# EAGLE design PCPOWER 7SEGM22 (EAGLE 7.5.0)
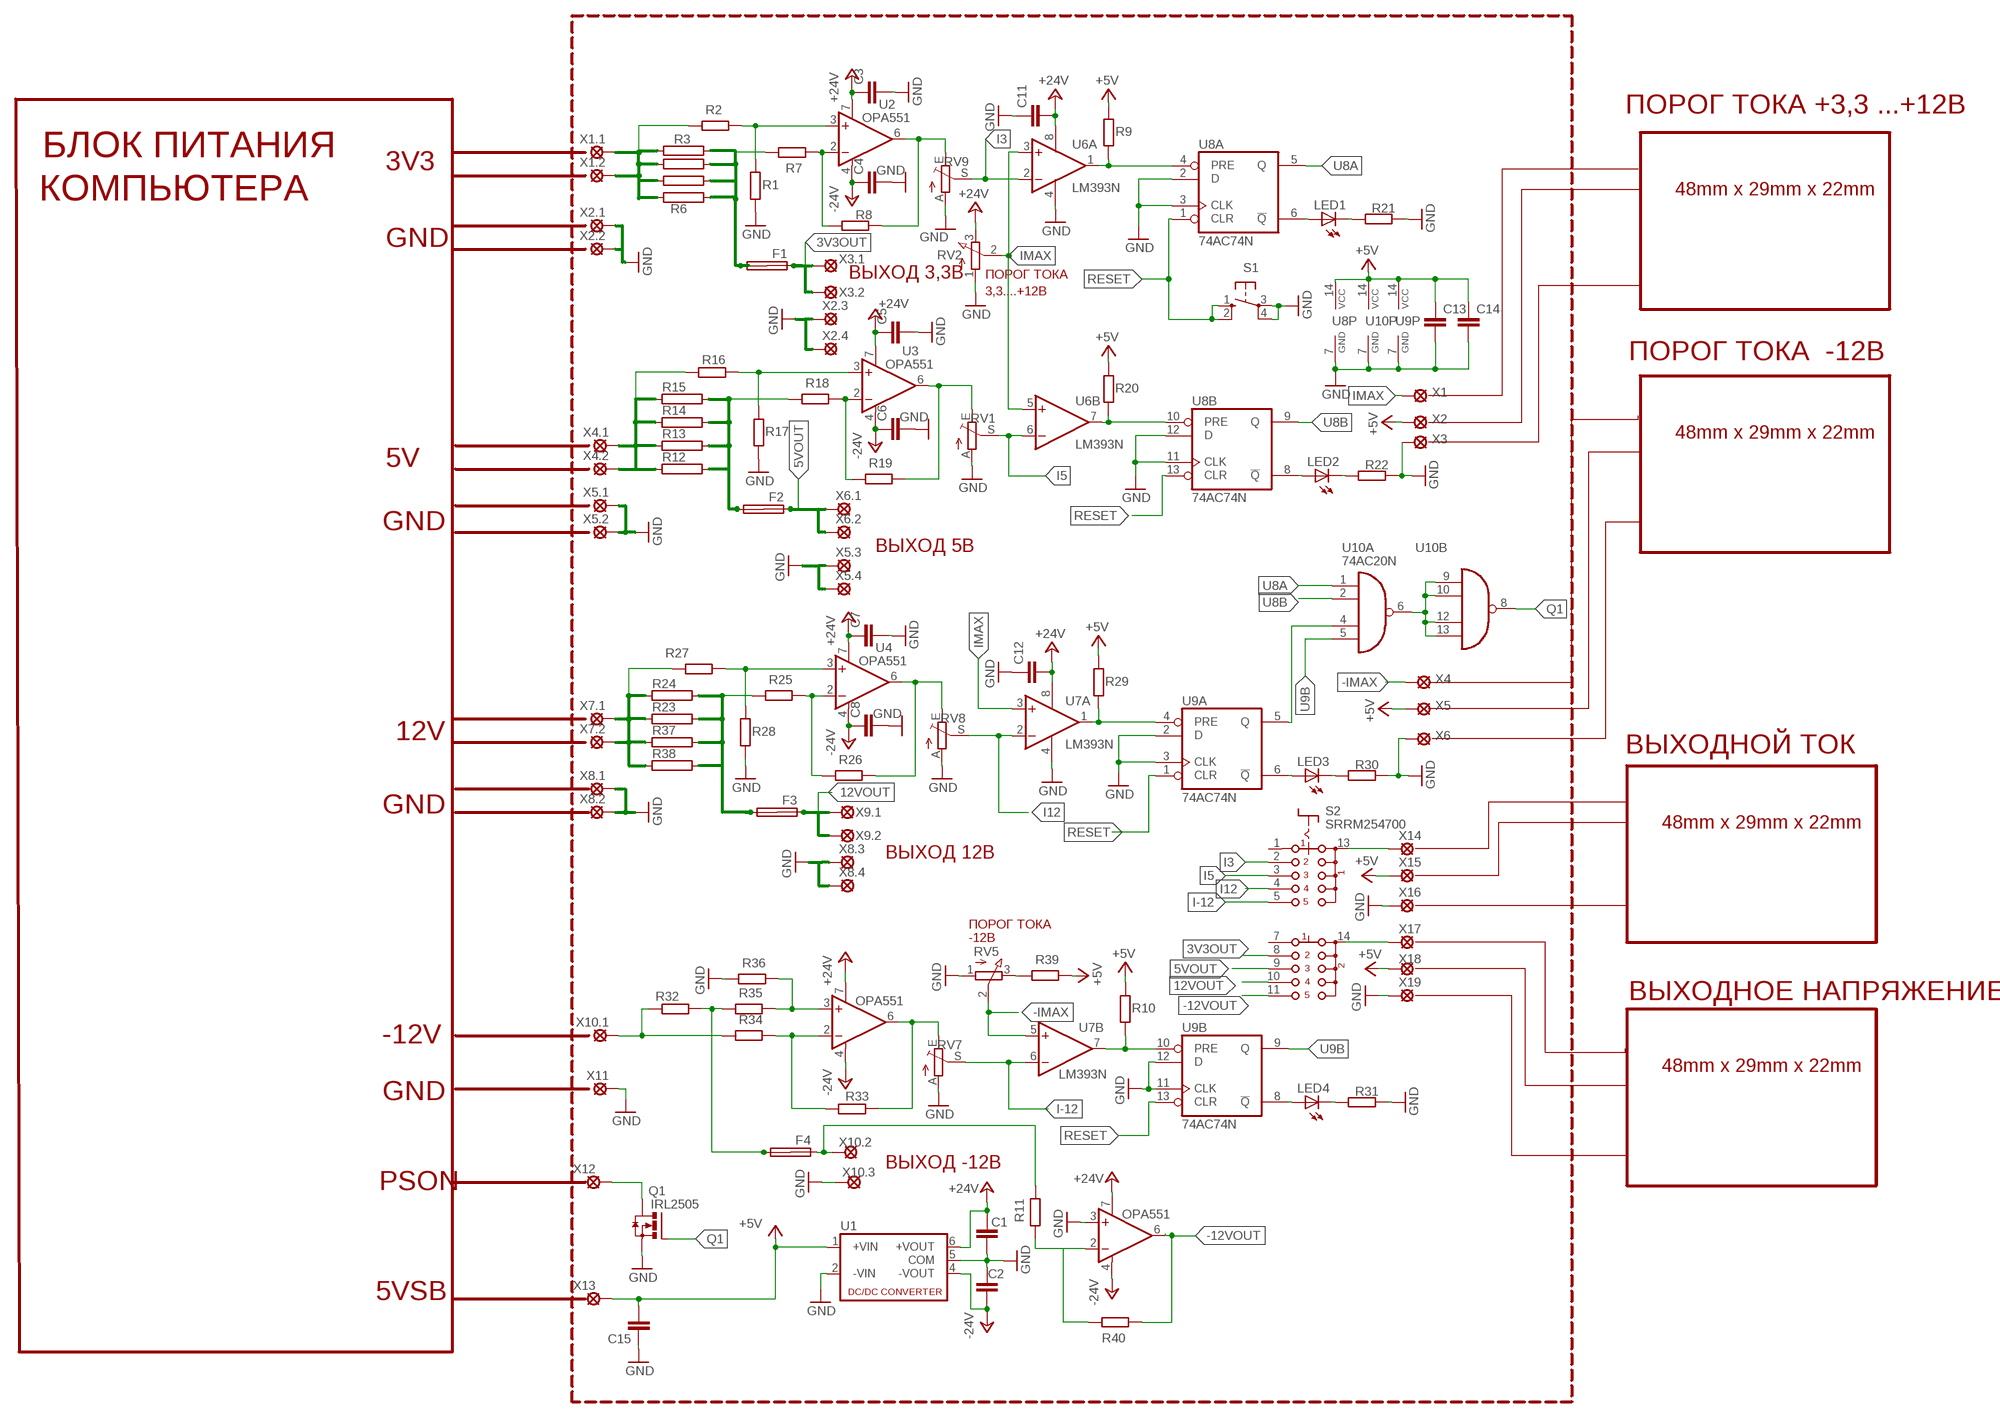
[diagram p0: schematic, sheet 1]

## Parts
C1  C-EUC1206  [C1206]
C2  C-EUC1206  [C1206]
C3  C-EUC1206  [C1206]
C4  C-EUC1206  [C1206]
C5  C-EUC1206  [C1206]
C6  C-EUC1206  [C1206]
C7  C-EUC1206  [C1206]
C8  C-EUC1206  [C1206]
C11  C-EUC1206  [C1206]
C12  C-EUC1206  [C1206]
C13  C-EUC1206  [C1206]
C14  C-EUC1206  [C1206]
C15  C-EUC1206  [C1206]
F1  SHK20L  [SHK20L]
F2  SHK20L  [SHK20L]
F3  SHK20L  [SHK20L]
F4  SHK20L  [SHK20L]
LED1  LED5MM  [LED5MM]
LED2  LED5MM  [LED5MM]
LED3  LED5MM  [LED5MM]
LED4  LED5MM  [LED5MM]
Q1  IRL2505  IRF3704L-V  [TO262-V]
R1  R-EU_0204/7  [0204/7]
R2  R-EU_0204/7  [0204/7]
R3  RKH208-8  [KH208-8]
R4  RKH208-8  [KH208-8]
R5  RKH208-8  [KH208-8]
R6  RKH208-8  [KH208-8]
R7  R-EU_0204/7  [0204/7]
R8  R-EU_0204/7  [0204/7]
R9  R-EU_0204/7  [0204/7]
R10  R-EU_0204/7  [0204/7]
R11  R-EU_0204/7  [0204/7]
R12  RKH208-8  [KH208-8]
R13  RKH208-8  [KH208-8]
R14  RKH208-8  [KH208-8]
R15  RKH208-8  [KH208-8]
R16  R-EU_0204/7  [0204/7]
R17  R-EU_0204/7  [0204/7]
R18  R-EU_0204/7  [0204/7]
R19  R-EU_0204/7  [0204/7]
R20  R-EU_0204/7  [0204/7]
R21  R-EU_0204/7  [0204/7]
R22  R-EU_0204/7  [0204/7]
R23  RKH208-8  [KH208-8]
R24  RKH208-8  [KH208-8]
R25  R-EU_0204/7  [0204/7]
R26  R-EU_0204/7  [0204/7]
R27  R-EU_0204/7  [0204/7]
R28  R-EU_0204/7  [0204/7]
R29  R-EU_0204/7  [0204/7]
R30  R-EU_0204/7  [0204/7]
R31  R-EU_0204/7  [0204/7]
R32  R-EU_0617/22  [0617/22]
R33  R-EU_0204/7  [0204/7]
R34  R-EU_0204/7  [0204/7]
R35  R-EU_0204/7  [0204/7]
R36  R-EU_0204/7  [0204/7]
R37  RKH208-8  [KH208-8]
R38  RKH208-8  [KH208-8]
R39  R-EU_0204/7  [0204/7]
R40  R-EU_0204/7  [0204/7]
RV1  TRIM_EU-CT6  [CT6]
RV2  PV09A  [PTV09]
RV5  PV09A  [PTV09]
RV7  TRIM_EU-CT6  [CT6]
RV8  TRIM_EU-CT6  [CT6]
RV9  TRIM_EU-CT6  [CT6]
S1  10-XX  [B3F-10XX]
S2  SRRM254700  [SRRM254700]
U1  NMA  [NMA]
U2  OPA551  OPA336P  [DIL08]
U3  OPA551  OPA336P  [DIL08]
U4  OPA551  OPA336P  [DIL08]
U5  OPA551  OPA336P  [DIL08]
U6  LM393N  [DIL08]
U7  LM393N  [DIL08]
U8  74AC74N  [DIL14]
U9  74AC74N  [DIL14]
U10  74AC20N  [DIL14]
U11  OPA551  OPA336P  [DIL08]
X1  LSP10  [LSP10]
X1.1  SE14  [SE14]
X1.2  SE14  [SE14]
X2  LSP10  [LSP10]
X2.1  SE14  [SE14]
X2.2  SE14  [SE14]
X2.3  SE14  [SE14]
X2.4  SE14  [SE14]
X3  LSP10  [LSP10]
X3.1  SE14  [SE14]
X3.2  SE14  [SE14]
X4  LSP10  [LSP10]
X4.1  SE14  [SE14]
X4.2  SE14  [SE14]
X5  LSP10  [LSP10]
X5.1  SE14  [SE14]
X5.2  SE14  [SE14]
X5.3  SE14  [SE14]
X5.4  SE14  [SE14]
X6  LSP10  [LSP10]
X6.1  SE14  [SE14]
X6.2  SE14  [SE14]
X7.1  SE14  [SE14]
X7.2  SE14  [SE14]
X8.1  SE14  [SE14]
X8.2  SE14  [SE14]
X8.3  SE14  [SE14]
X8.4  SE14  [SE14]
X9.1  SE14  [SE14]
X9.2  SE14  [SE14]
X10.1  SE14  [SE14]
X10.2  SE14  [SE14]
X10.3  SE14  [SE14]
X11  SE14  [SE14]
X12  SE14  [SE14]
X13  SE14  [SE14]
X14  LSP10  [LSP10]
X15  LSP10  [LSP10]
X16  LSP10  [LSP10]
X17  LSP10  [LSP10]
X18  LSP10  [LSP10]
X19  LSP10  [LSP10]

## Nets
3V3OUT: F1.1A S2.8 X3.1.MP X3.2.MP
5VOUT: F2.1A S2.9 X6.1.MP X6.2.MP
12VOUT: F3.1A S2.10 X9.1.MP X9.2.MP
+5V: C13.1 C14.1 C15.2 R9.2 R10.2 R20.2 R29.2 R39.1 U1.1(+VIN) U8.14(P:VCC) U9.14(P:VCC) U10.14(P:VCC) X2.MP X5.MP X13.MP X15.MP X18.MP
+24V: C1.1 C3.1 C5.1 C7.1 C11.2 C12.2 RV2.3(E) U1.6(+VOUT) U2.7(V+) U3.7(V+) U4.7(V+) U5.7(V+) U6.8(P:V+) U7.8(P:V+) U11.7(V+)
-12VOUT: R40.2 S2.11
-24V: C2.2 C4.1 C6.1 C8.1 U1.4(-VOUT) U2.4(V-) U3.4(V-) U4.4(V-) U5.4(V-) U11.4(V-)
-IMAX: RV5.2(S) U7.5(B:+IN) X4.MP
GND: C1.2 C2.1 C3.2 C4.2 C5.2 C6.2 C7.2 C8.2 C11.1 C12.1 C13.2 C14.2 C15.1 Q1.3(S) R1.1 R17.1 R21.2 R22.2 R28.1 R30.2 R31.2 R36.2 RV1.A RV2.1(A) RV5.1(A) RV7.A RV8.A RV9.A S1.3(P) S1.4(P1) U1.2(-VIN) U1.5(COM) U6.4(P:V-) U7.4(P:V-) U8.2(A:D) U8.3(A:CLK) U8.7(P:GND) U8.11(B:CLK) U8.12(B:D) U9.2(A:D) U9.3(A:CLK) U9.7(P:GND) U9.11(B:CLK) U9.12(B:D) U10.7(P:GND) U11.3(+IN) X2.1.MP X2.2.MP X2.3.MP X2.4.MP X3.MP X5.1.MP X5.2.MP X5.3.MP X5.4.MP X6.MP X8.1.MP X8.2.MP X8.3.MP X8.4.MP X10.3.MP X11.MP X16.MP X19.MP
I3: RV9.S S2.2 U6.2(A:-IN)
I5: RV1.S S2.3 U6.6(B:-IN)
I12: RV8.S S2.4 U7.2(A:-IN)
I-12: RV7.S S2.5 U7.6(B:-IN)
IMAX: RV2.2(S) U6.3(A:+IN) U6.5(B:+IN) U7.3(A:+IN) X1.MP
N$1: R1.2 R2.1 U2.3(+IN)
N$2: R7.2 R8.1 U2.2(-IN)
N$3: R8.2 RV9.E U2.6(OUT)
N$4: R23.1 R24.1 R27.2 R37.1 R38.1 X7.1.MP X7.2.MP
N$5: R9.1 U6.1(A:OUT) U8.4(A:PRE)
N$6: R12.1 R13.1 R14.1 R15.1 R16.2 X4.1.MP X4.2.MP
N$7: F2.2A R12.2 R13.2 R14.2 R15.2 R18.2
N$8: R16.1 R17.2 U3.3(+IN)
N$9: R18.1 R19.2 U3.2(-IN)
N$10: R19.1 RV1.E U3.6(OUT)
N$11: F3.2A R23.2 R24.2 R25.2 R37.2 R38.2
N$12: R27.1 R28.2 U4.3(+IN)
N$13: R25.1 R26.2 U4.2(-IN)
N$14: R26.1 RV8.E U4.6(OUT)
N$15: R20.1 U6.7(B:OUT) U8.10(B:PRE)
N$16: R29.1 U7.1(A:OUT) U9.4(A:PRE)
N$17: R32.1 R34.2 X10.1.MP
N$18: R33.2 R34.1 U5.2(-IN)
N$19: R33.1 RV7.E U5.6(OUT)
N$20: F4.2A R32.2 R35.2
N$21: R35.1 R36.1 U5.3(+IN)
N$22: R39.2 RV5.3(E)
N$23: F4.1A R11.1 X10.2.MP
N$24: R10.1 U7.7(B:OUT) U9.10(B:PRE)
N$25: S2.13(C1) X14.MP
N$26: S2.14(C2) X17.MP
N$27: R11.2 R40.1 U11.2(-IN)
N$29: LED1.A U8.6(A:!Q)
N$30: LED1.K(C) R21.1
N$31: LED2.A U8.8(B:!Q)
N$32: LED2.K(C) R22.1
N$33: Q1.2(D) X12.MP
N$35: LED3.A U9.6(A:!Q)
N$37: LED3.K(C) R30.1
N$38: LED4.A U9.8(B:!Q)
N$39: LED4.K(C) R31.1
N$40: U9.5(A:Q) U10.4(A:I2)
N$42: U10.6(A:O) U10.9(B:I0) U10.10(B:I1) U10.12(B:I2) U10.13(B:I3)
N$44: F1.2A R3.2 R4.2 R5.2 R6.2 R7.1
N$45: R2.2 R3.1 R4.1 R5.1 R6.1 X1.1.MP X1.2.MP
Q1: Q1.1(G) U10.8(B:O)
RESET: S1.1(S) S1.2(S1) U8.1(A:CLR) U8.13(B:CLR) U9.1(A:CLR) U9.13(B:CLR)
U8A: U8.5(A:Q) U10.1(A:I0)
U8B: U8.9(B:Q) U10.2(A:I1)
U9B: U9.9(B:Q) U10.5(A:I3)
Unconnected: F1.1B F1.2B F2.1B F2.2B F3.1B F3.2B F4.1B F4.2B S2.1 S2.7 U11.6(OUT)

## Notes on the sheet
- ПОРОГ ТОКА +3,3 ...+12В
- БЛОК ПИТАНИЯ
- 3V3
- КОМПЬЮТЕРА | 48mm x 29mm x 22mm
- GND
- ВЫХОД 3,3В | ПОРОГ ТОКА
- 3,3....+12В
- ПОРОГ ТОКА  -12В
- 48mm x 29mm x 22mm
- 5V
- GND
- ВЫХОД 5В
- 12V
- ВЫХОДНОЙ ТОК
- GND
- 48mm x 29mm x 22mm
- ВЫХОД 12В
- ПОРОГ ТОКА
- -12В
- ВЫХОДНОЕ НАПРЯЖЕНИЕ
- -12V
- 48mm x 29mm x 22mm
- GND
- ВЫХОД -12В
- PSON
- 5VSB

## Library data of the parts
C1-C8 C11-C15 = rcl:C-EU: CAPACITOR, European symbol
F1-F4 = fuse:SHK20L: FUSE HOLDER 5 x 20 mm, SH contact, SHH1 Schukat, E1073 Buerklin; OC_FARNELL: unknown; OC_NEWARK: unknown
LED1-LED4 = led:LED: LED
Q1 = transistor-power:IRF3704: SMPS MOSFET HEXFET® Power MOSFET Source: http://www.irf.com/product-info/datasheets/data/irf3704.pdf
R1 R2 R7-R11 R16-R22 R25-R36 R39 R40 = rcl:R-EU_: RESISTOR, European symbol
R3-R6 R12-R15 R23 R24 R37 R38 = resistor-power:R: Power Resitor; OC_FARNELL: unknown; OC_NEWARK: unknown
RV1 RV7-RV9 = pot:TRIM_EU-: POTENTIOMETER
RV2 RV5 = pot:PV09A
S1 = switch-omron:10-XX: OMRON SWITCH; MPN: B3F-1000; OC_FARNELL: 176432; OC_NEWARK: 36M3542
S2 = switch:SRRM254700: 12-position General-purpose Vertical Type Rotary Switch 2 Pole 5 Positions Source: ALPS - SRRM.pdf
U1 = dc-dc-converter:NMA: DC-DC CONVERTER; MF: C & D TECHNOLOGIES, INC; MPN: NMA0515SC; OC_FARNELL: 1021434; OC_NEWARK: 61K3064
U2-U5 U11 = burr-brown:OPA336: CMOS Operational Amplifiers Single-Supply, MicroPower, MicroAmplifier(TM) Series; OC_FARNELL: unknown; OC_NEWARK: unknown
U6 U7 = linear:LM393: COMPARATOR
U8 U9 = 74xx-eu:74*74: Dual D type positive edge triggered FLIP FLOP, preset and clear
U10 = 74xx-eu:74*20: Dual 4-input NAND gate
X1-X6 X14-X19 = solpad:LSP10: SOLDER PAD
X1.1 X1.2 X2.1-X2.4 X3.1 X3.2 X4.1 X4.2 X5.1-X5.4 X6.1 X6.2 X7.1 X7.2 X8.1-X8.4 X9.1 X9.2 X10.1-X10.3 X11-X13 = solpad:SE14: SOLDER PAD

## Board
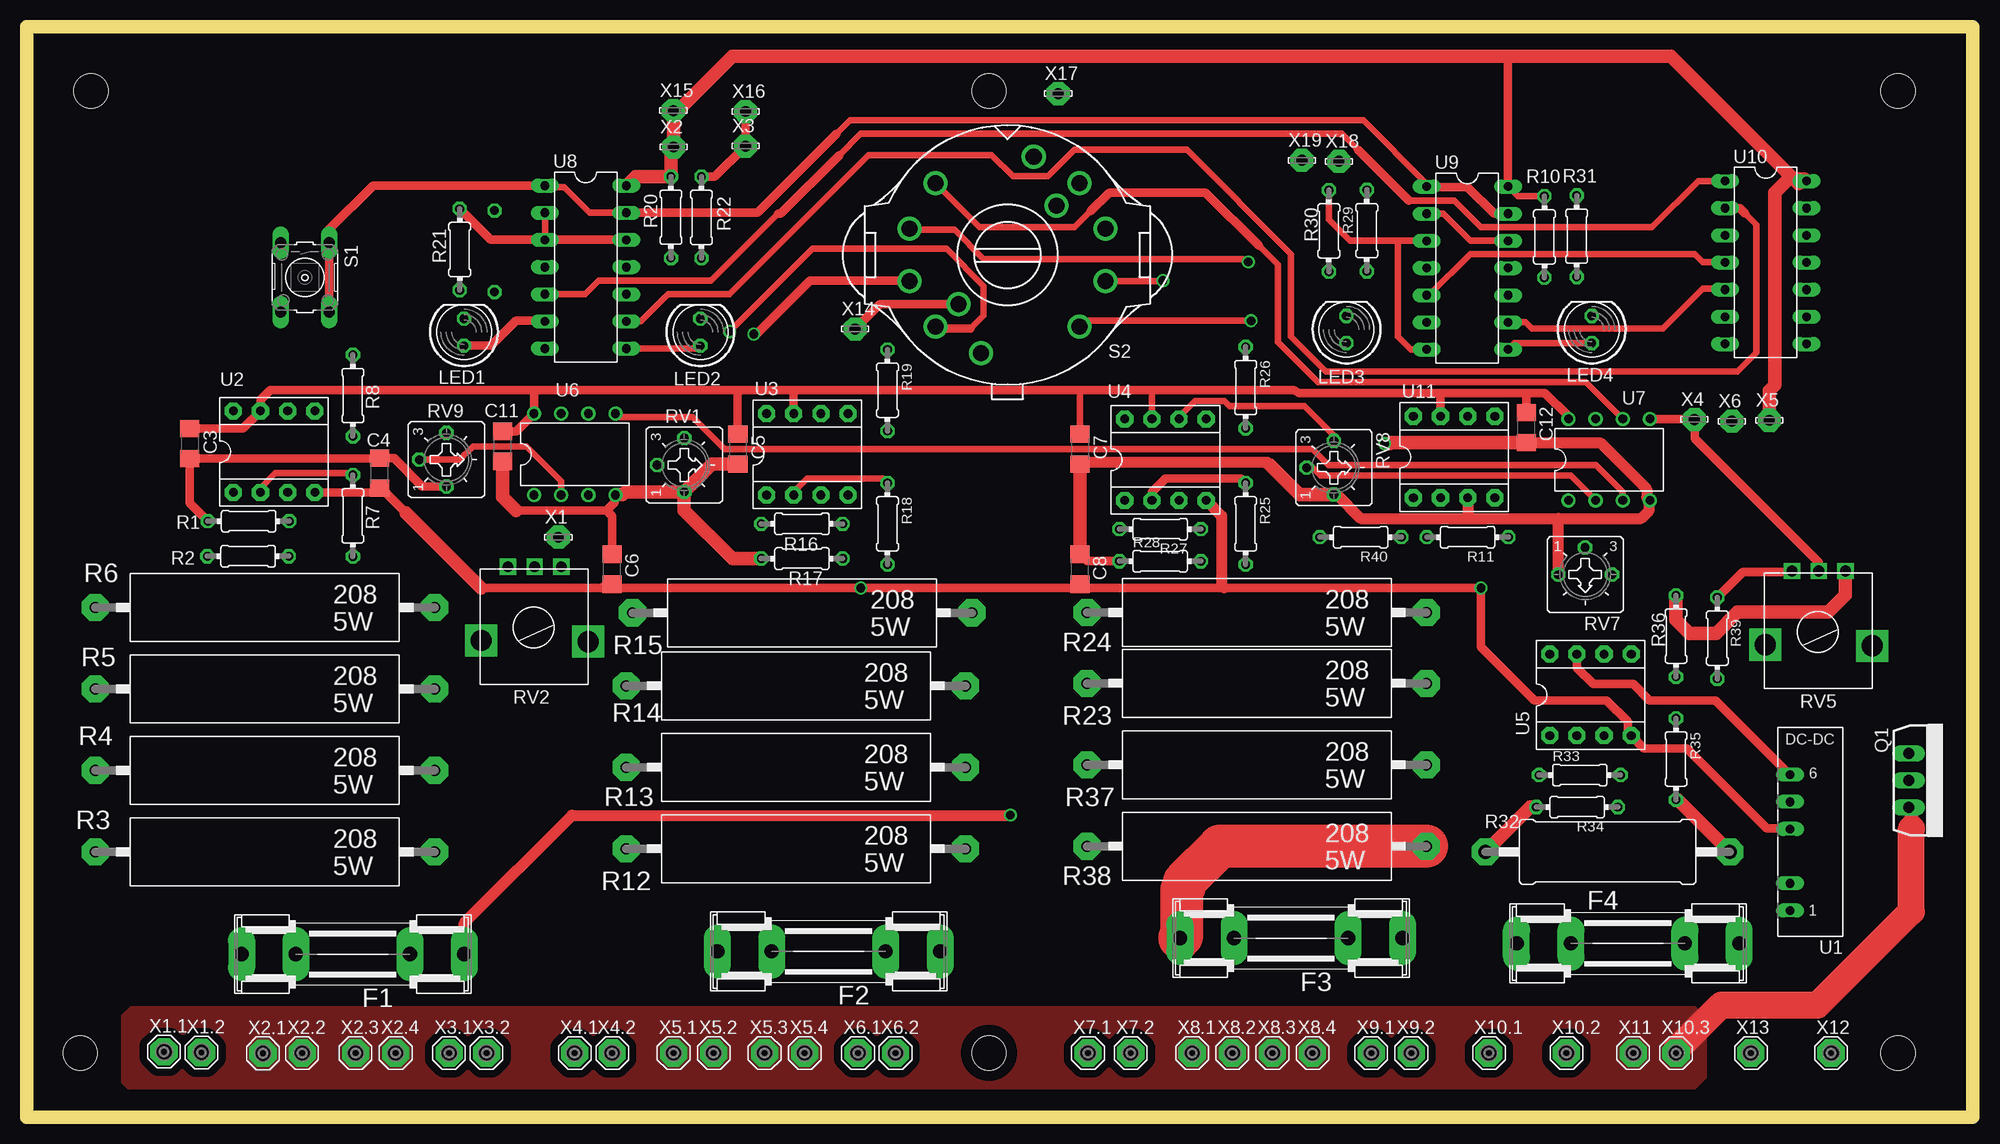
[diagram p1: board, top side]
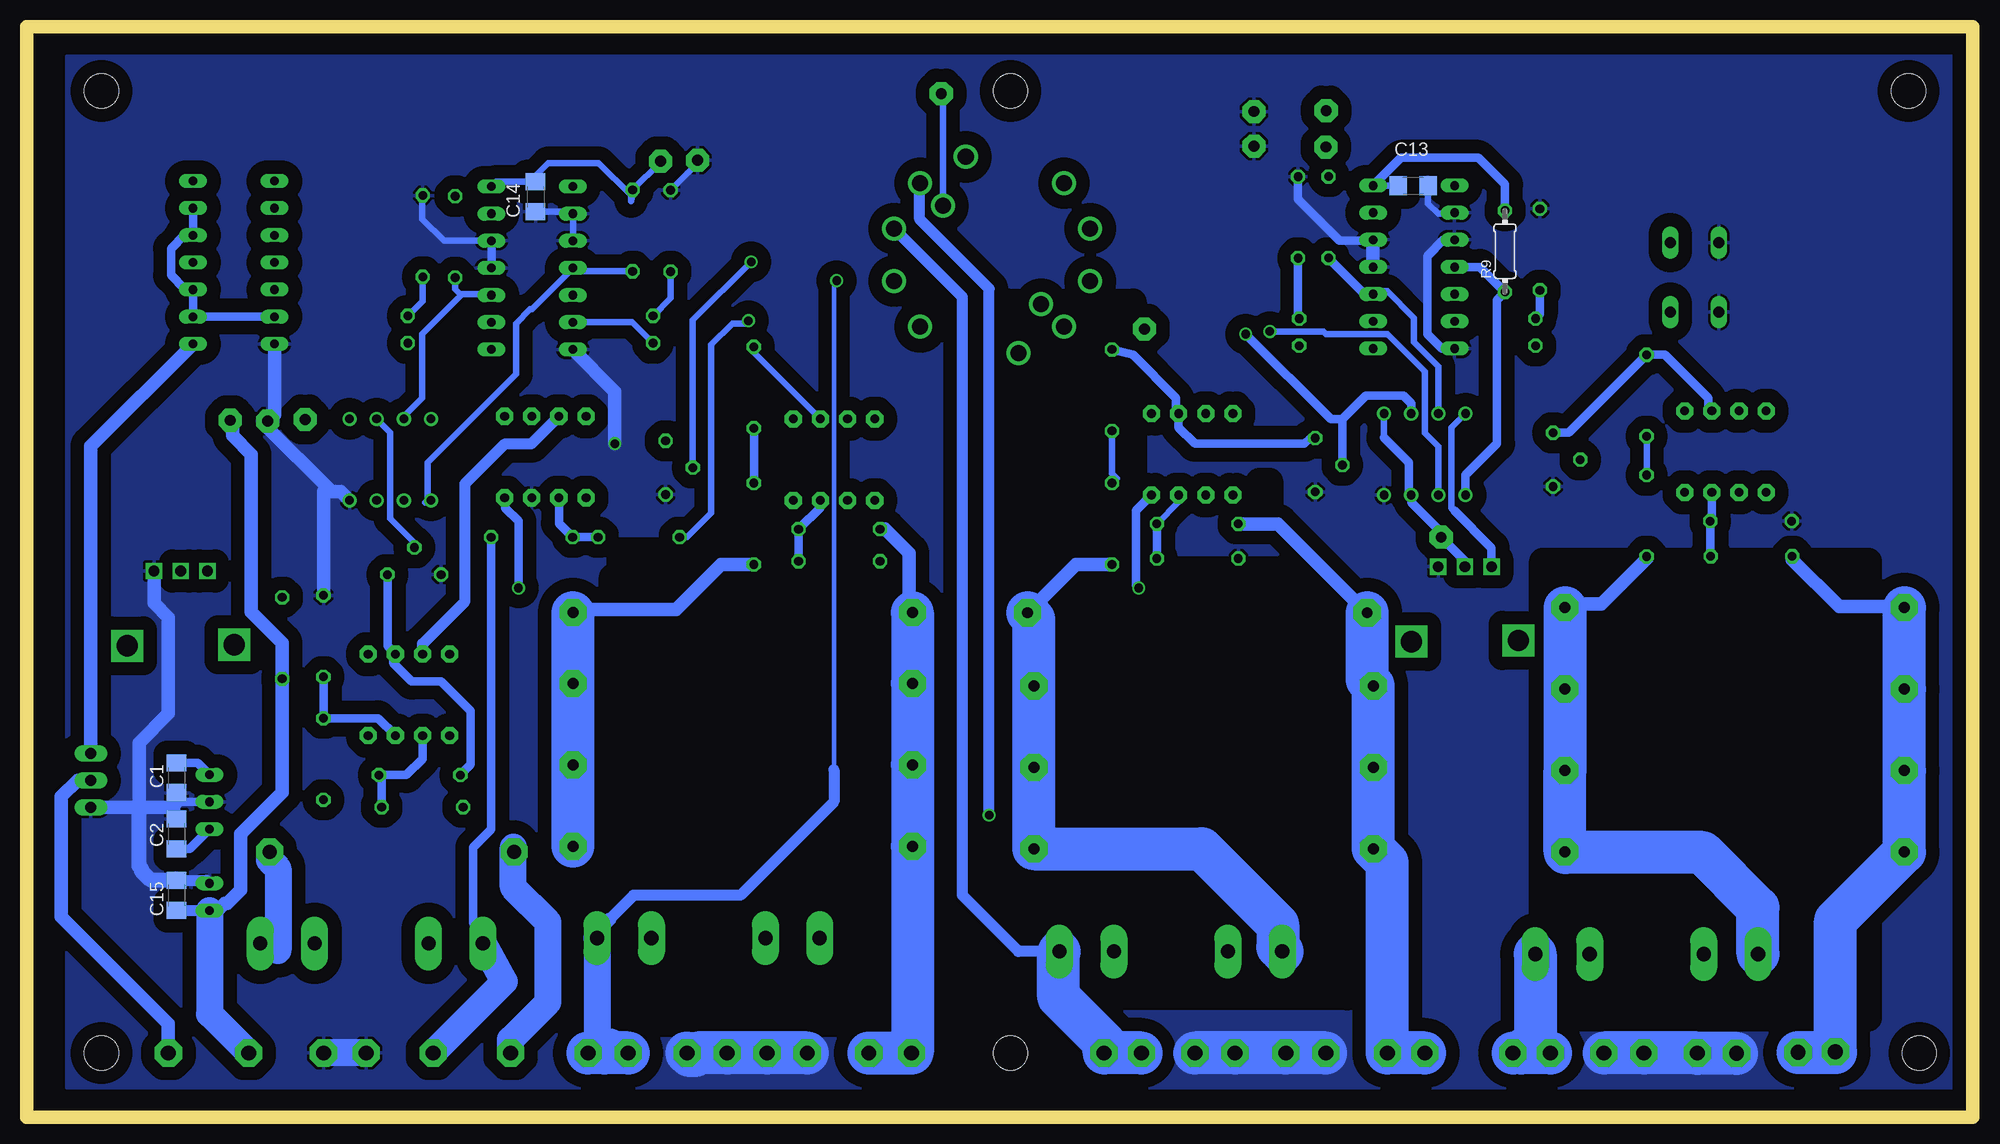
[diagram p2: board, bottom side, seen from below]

Size 182 x 102 mm. Coordinates in mm from the lower left corner, seen from the top.
Outline: 0,102 182,102 182,0 0,0 0,102
Copper layers (1*16): Top 0.035mm / dielectric 1.5mm / Bottom 0.035mm
Design rules "default": minimum track width 10mil, minimum drill 24mil, track to track 8mil, track to pad 8mil, pad to pad 8mil, via to via 8mil, smd to smd 8mil, copper to edge 40mil, drill to drill 8mil, minimum pad ring 10mil, minimum via ring 8mil, stop-mask expansion 4mil, vias tented up to drill 0mil, thermal gap 10mil
Holes 3.2 mm at 5,6 90,6 175,6 175,96 90,96 6,96
bRestrict: area 63.2,47 to 63.5,48.5; area 64.8,34 to 80.5,51.2; area 59.5,29 to 64.8,50.5; area 58.8,28.2 to 85.5,36; area 58.5,11.2 to 94,27.2; area 9.8,9.2 to 40.2,52; area 78.5,50.5 to 90.2,76.2; area 101.8,50.2 to 102,51.5; area 107.2,24 to 127.2,50.5; area 100,8.8 to 126.5,53; area 65.8,57.5 to 66.8,59.5

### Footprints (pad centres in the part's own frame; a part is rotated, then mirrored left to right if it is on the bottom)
C1206 = smd 1.6 x 1.8: 1 -1.4,0; 2 1.4,0
SHK20L = drill 1.321 pad 2.54 long: 1A -10.414,0; 1B -5.334,0; 2A 10.414,0; 2B 5.334,0
LED5MM = drill 0.813 octagon: A -1.27,0; K 1.27,0
TO262-V = drill 1.016 long: 1 -2.54,0; 2 0,0; 3 2.54,0
0204/7 = drill 0.813 octagon: 1 -3.81,0; 2 3.81,0
KH208-8 = drill 1.016 pad 2.54 octagon: 1 -15.875,0; 2 15.875,0
0617/22 = drill 1.3 pad 2.54 octagon: 1 -11.43,0; 2 11.43,0
CT6 = drill 0.813 octagon: A 2.515,0; E -2.515,0; S 0,-2.54
PTV09 = drill 1 square: 1 -2.5,0; 2 0,0; 3 2.5,0 | drill 2 square: P$4 -5,7; P$5 5,6.9
B3F-10XX = drill 1.016 long: 1 -3.251,2.261; 2 3.251,2.261; 3 -3.251,-2.261; 4 3.251,-2.261
SRRM254700 = drill 1.5 pad 2.184: 1 -9.176,2.459; 2 -6.718,6.718; 3 -2.459,9.176; 4 2.459,9.176; 5 6.718,6.718; 7 9.176,-2.459; 8 6.718,-6.718; 9 2.459,-9.176; 10 -2.459,-9.176; 11 -6.718,-6.718; 13 -4.596,4.596; 14 4.596,-4.596
NMA = drill 0.813 long: 1 0,6.35; 2 0,3.81; 4 0,-1.27; 5 0,-3.81; 6 0,-6.35
DIL08 = drill 0.813 pad 1.6 octagon: 1 -3.81,-3.81; 2 -1.27,-3.81; 3 1.27,-3.81; 4 3.81,-3.81; 5 3.81,3.81; 6 1.27,3.81; 7 -1.27,3.81; 8 -3.81,3.81
DIL08' = drill 0.813 pad 1.27: 1 -3.81,-3.81; 2 -1.27,-3.81; 3 1.27,-3.81; 4 3.81,-3.81; 5 3.81,3.81; 6 1.27,3.81; 7 -1.27,3.81; 8 -3.81,3.81
DIL14 = drill 0.813 long: 1 -7.62,-3.81; 2 -5.08,-3.81; 3 -2.54,-3.81; 4 0,-3.81; 5 2.54,-3.81; 6 5.08,-3.81; 7 7.62,-3.81; 8 7.62,3.81; 9 5.08,3.81; 10 2.54,3.81; 11 0,3.81; 12 -2.54,3.81; 13 -5.08,3.81; 14 -7.62,3.81
LSP10 = drill 1.016 pad 2.159 octagon: MP 0,0
SE14 = drill 1.397 pad 2.54 octagon: MP 0,0

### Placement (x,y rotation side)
C1  168,31.75 270 bottom
C2  168,26.5 270 bottom
C3  15.25,63 270 top
C4  33,60.25 90 top
C5  66.5,62.5 270 top
C6  54.75,51.25 90 top
C7  98.5,62.5 270 top
C8  98.5,51.25 90 top
C11  44.5,62.75 90 top
C12  140.25,64.5 90 top
C13  52.34,87.14 0 bottom
C14  134.42,86.09 270 bottom
C15  168,20.75 270 bottom
F1  30.5,15.25 180 top
F2  75,15.5 180 top
F3  118.25,16.75 180 top
F4  149.75,16.25 0 top
LED1  40.89,73.43 90 top
LED2  63,73.43 90 top
LED3  123.43,73.68 90 top
LED4  146.36,73.68 90 top
Q1  176,31.5 270 top
R1  20.75,55.75 0 top
R2  20.7,52.47 180 top
R3  22.27,24.81 0 top
R4  22.27,32.43 0 top
R5  22.27,40.05 0 top
R6  22.27,47.67 0 top
R7  30.5,56.25 90 top
R8  30.5,67.5 90 top
R9  43.75,81 90 bottom
R10  141.94,82.34 90 top
R11  134.75,54.25 180 top
R12  71.93,25.11 0 top
R13  71.93,32.73 0 top
R14  71.93,40.35 0 top
R15  72.52,47.18 0 top
R16  72.5,55.5 180 top
R17  72.5,52.25 0 top
R18  80.5,55.5 270 top
R19  80.5,68 270 top
R20  60.25,84.18 90 top
R21  40.49,81.16 90 top
R22  63.1,84.16 90 top
R23  115.04,40.58 0 top
R24  115.04,47.2 0 top
R25  114,55.5 270 top
R26  114,68.25 270 top
R27  106,55 180 top
R28  106,52 0 top
R29  125.33,82.93 90 top
R30  121.78,82.91 90 top
R31  144.96,82.41 90 top
R32  147.86,24.82 0 top
R33  145.25,32 0 top
R34  145,29 180 top
R35  154.25,33.5 270 top
R36  154.25,45 90 top
R37  115.04,32.96 0 top
R38  115.04,25.34 0 top
R39  158.11,44.81 90 top
R40  124.75,54.25 180 top
RV1  61.5,61 270 top
RV2  47.5,51.49 180 top
RV5  167.6,51.09 180 top
RV7  145.75,50.75 180 top
RV8  122.25,60.75 270 top
RV9  39.25,61.5 270 top
S1  26.02,78.55 270 top
S2  91.72,80.65 90 top
U1  164.91,25.68 180 top
U2  23.13,62.25 0 top
U3  73,62 0 top
U4  106.5,61.5 0 top
U5  146.25,39.5 0 top
U6  LM393N  [DIL08']  51.25,62 0 top
U7  LM393N  [DIL08']  148,61.5 0 top
U8  52.27,79.52 270 top
U9  134.73,79.43 270 top
U10  162.64,79.95 270 top
U11  133.5,61.75 0 top
X1  49.72,54.25 0 top
X1.1  12.84,6.13 0 top
X1.2  16.34,6.05 0 top
X2  60.5,90.75 0 top
X2.1  22.09,5.97 0 top
X2.2  25.75,6 0 top
X2.3  30.75,6 0 top
X2.4  34.5,6 0 top
X3  67.22,90.84 0 top
X3.1  39.5,6 0 top
X3.2  43,6 0 top
X4  155.97,65.26 0 top
X4.1  51.25,6 0 top
X4.2  54.75,6 0 top
X5  162.97,65.18 0 top
X5.1  60.5,6 0 top
X5.2  64.25,6 0 top
X5.3  69,6 0 top
X5.4  72.75,6 0 top
X6  159.47,65.1 0 top
X6.1  77.75,6 0 top
X6.2  81.25,6 0 top
X7.1  99.25,6 0 top
X7.2  103.25,6 0 top
X8.1  109,6 0 top
X8.2  112.75,6 0 top
X8.3  116.5,6 0 top
X8.4  120.25,6 0 top
X9.1  125.75,6 0 top
X9.2  129.5,6 0 top
X10.1  136.75,6 0 top
X10.2  144,6 0 top
X10.3  154.25,6 0 top
X11  150.25,6 0 top
X12  168.75,6 0 top
X13  161.25,6 0 top
X14  77.47,73.73 0 top
X15  60.47,94.15 0 top
X16  67.22,94.07 0 top
X17  96.47,95.74 0 top
X18  122.72,89.41 0 top
X19  119.25,89.5 0 top

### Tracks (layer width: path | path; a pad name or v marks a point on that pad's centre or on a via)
3V3OUT  (via drill 0.8)
  Top 1.016: F1.1A 40.91,18.16 51,28.25 v92,28.25
  Bottom 1.016: v92,28.25 92,77.5 98.5,84 98.5,87.31 S2.8
  Bottom 4: X3.1.MP 42.25,6 | 42.25,6 X3.2.MP | F1.1A 40.91,7.34 42.25,6
5VOUT
  Bottom 1.016: F2.1A 89.25,15.5 94.5,20.75 94.5,76.71 S2.9
  Bottom 4: X6.1.MP X6.2.MP 81.25,7 85.5,11.25 85.5,15.41 F2.1A
12VOUT  (via drill 0.8)
  Top 0.61: S2.10 106.19,78.19 v106.25,78.25
  Bottom 0.41: 106.5,78 106.5,32.5
  Bottom 0.61: v106.25,78.25 106.5,78
  Bottom 1.016: 106.5,32.5 106.5,29.5 115.25,20.75 125.25,20.75 127.5,18.5
  Bottom 1.27: 127.5,18.5 129.25,16.75 F3.1A
  Bottom 2.54: F3.1A 128.66,6.84 X9.2.MP
  Bottom 4: X9.1.MP 128,6 | 128,6 X9.2.MP | 127.66,6.34 128,6
+5V
  Top 0.61: R10.2 139.44,86.15 U9.14
  Top 0.813: U9.14 138.54,99.04 138.75,99.25
  Top 1.27: 60.5,94.12 60.87,94.12 66,99.25 138.75,99.25 153.75,99.25 165.68,87.32 U10.14 166.27,87.75 164.75,87.75 163.5,86.5 163.5,68.5 162.97,67.97 X5.MP | 60.5,94.12 X2.MP 60.25,90.5 R20.2 56.93,87.99 U8.14 | 60.5,94.12 X15.MP
  Bottom 0.61: C13.1 U8.14 | U9.14 138.1,87.49 C14.1 134.42,88.08 133.25,89.25 128.5,89.25 125.5,86.25 125.5,85.66 R29.2 122.72,89.35 X18.MP
  Bottom 0.813: 138.51,87.08 U9.14 | R9.2 43.75,87.25 46.25,89.75 53.47,89.75 U8.14
  Bottom 1.016: C15.2 164.93,19.35 U1.1
  Bottom 1.27: U1.1 164.74,19.5 164,19.5 163.5,20 163.25,20 162,21.25 162,26.5 158.11,30.39 R39.1 158.11,44.36 161,47.25 161,62 162.75,63.75 162.75,64.96 X5.MP
  Bottom 2.54: U1.1 164.91,9.66 X13.MP
+24V
  Top 0.61: U4.7 105.23,67.98 105.25,68 | C7.1 98.5,67.75 98.75,68
  Top 0.813: 47.25,68 22.75,68 21.86,67.11 U2.7 20.2,64.4 C3.1 | 47.25,68 66.5,68 | 66.5,68 71.5,68 | 71.5,68 98.75,68 105.25,68 118.5,68 119,67.75 132,67.75 | 47.25,68 47.44,67.81 U6.8 45.78,64.15 C11.2 | U3.7 71.73,67.77 71.5,68 | C5.1 66.5,68 | 132,67.75 140.5,67.75 | 140.5,67.75 142,67.75 144.19,65.56 U7.8 | U11.7 132.23,67.52 132,67.75 | C12.2 140.25,67.5 140.5,67.75 | U5.7 144.98,42.02 146.5,40.5 150.25,40.5 151.75,39 157.94,39 U1.6
  Bottom 0.61: 48.5,56.75 48.75,57 48.75,64.5 U6.8
  Bottom 0.813: RV2.3 45,53.25 48.5,56.75 | C1.1 166.03,33.15 U1.6
  Bottom 1.016: U5.7 144.98,44.27 141,48.25 141,59.25 137.25,63 134.79,63 U11.7
-12VOUT  (via drill 0.8)
  Top 0.61: v114.5,74.5 99,74.5 S2.11
  Bottom 0.61: R40.2 120.25,54.25 118,56.5 118,72.25 116,74.25 114.75,74.25 v114.5,74.5
-24V  (via drill 0.8)
  Top 0.813: U2.4 32.59,58.44 C4.1 33.15,58.85 35.5,56.5 | 42.5,49.5 53.75,49.5 | 53.75,49.5 v78,49.5 98.75,49.5 | 98.75,49.5 112,49.5 v136,49.5 136,44 141,39 147.75,39 149.75,37 149.75,36 U5.4 151.25,34.5 155.25,34.5 162.75,27 164.86,27 U1.4 | C6.1 53.85,49.6 53.75,49.5 | 98.75,49.5 98.5,49.75 C8.1
  Top 1.016: U4.4 111.75,56.25 111.75,49.75 112,49.5
  Top 1.27: 35.5,56.5 42.5,49.5
  Bottom 0.813: U3.4 78.25,56.75 78.25,49.75 v78,49.5 | v136,49.5 136,55.75 137.25,57 137.25,57.88 U11.4 | C2.2 166.76,25.1 U1.4
-IMAX
  Top 0.813: RV5.2 167.6,51.9 156,63.5 156,65.23 X4.MP 155.92,65.31 U7.5
GND  (via drill 0.8)
  Top 0.61: U9.12 135.03,81.97 132.5,84.5 U9.2 | U9.7 129.44,71.81 128.25,73 128.25,82 | U8.3 U8.2 | R30.2 121.78,83.97 123.75,82 128.25,82 | 128.25,82 130.89,82 U9.3
  Top 0.813: R1.1 15.25,57.44 C3.2 32.95,61.6 C4.2 34.35,61.65 37,59 39.23,59 RV9.A | R28.1 99.15,52 C8.2 | U8.12 U8.3 43.4,82.06 R21.2 | X16.MP X3.MP 64.35,87.97 R22.2 | 45.75,56.75 54.25,56.75 | 54.25,56.75 55,57.5 55,58.13 U6.4 | C6.2 54.75,56.25 54.25,56.75
  Top 1.016: 116.25,61 116,61.25 98.65,61.25 C7.2 | RV8.A 122.52,58.23 124.75,56 135,56 | 135,56 143.25,56 | 143.25,56 151,56 151.75,56.75 151.75,57.63 U7.4 151.5,58 151.5,58.75 147.15,63.1 C12.1 | RV7.A 143.24,55.98 143.25,56 | U11.3 134.77,56.23 135,56
  Top 1.27: C5.2 64.11,61.1 RV1.A | RV1.A 55.98,58.48 55.75,58.25 55.12,58.25 U6.4 | RV8.A 119.02,58.23 116.25,61 | C12.1 127.6,63.1 | 127.5,63 v127,63 | RV5.1 170.1,48.85 168.5,47.25 160,47.25 158,45.25 155.5,45.25 154.25,46.5 R36.2 | 176.25,27 176.25,28.71 Q1.3 | R17.1 66,52.25 61.5,56.75 RV1.A | C11.1 44.5,58 45.75,56.75 | C7.2 C8.2
  Top 2.54: X10.3.MP 154.25,6.25 158.5,10.5 167.5,10.5 176.25,19.25 176.25,27
  Bottom 0.61: U9.3 U9.2 131.1,84.69 C14.2 | C13.2 50.94,85.44 50,84.5 48.56,84.5 U8.2 | U9.12 142.97,81.97 145,84 145,86.18 R31.2 | X19.MP 119.25,89.25 R30.2
  Bottom 0.813: U8.7 49.65,71.9 51,73.25 51,80.56 49.5,82.06 U8.3 | R22.2 63.1,85.85 59.25,82 56.14,82 U8.12 | C2.1 168,29.5 | 168,29.5 C1.2 | U1.5 167.99,29.49 168,29.5 | U9.11 U9.12
  Bottom 1.016: C15.1 165.19,22.15 U1.2
  Bottom 1.27: U8.11 U8.12 | v127,63 127,67.89 U9.7 | Q1.3 171.5,28.96 171.25,28.96 | 171.25,28.96 168.52,28.96 167.99,29.49 | 153.88,58.88 159.47,64.47 X6.MP 158.83,65.74 U10.7 | 153.88,58.88 153.5,58.5 152.62,58.5 U7.4 | R36.2 154.25,58.5 153.88,58.88 | RV5.1 170.1,48.1 168.75,46.75 168.75,37.75 171.5,35 171.5,29.21 171.25,28.96
  Bottom 1.422: C15.1 170.4,22.15 171.25,23 171.25,23.25 171.5,23.5 171.5,28.96
  Bottom 2.54: X11.MP X10.3.MP
  Bottom 4: X2.1.MP 25.72,5.97 X2.2.MP X2.3.MP X2.4.MP | X5.1.MP X5.2.MP X5.3.MP X5.4.MP | X8.1.MP X8.2.MP X8.3.MP 119.25,6 119.5,5.75 120,5.75 X8.4.MP
  pour Top (isolate 1.016, no thermals): 9.75,10.25 156,10.25 157,9.25 157,3.75 156,2.75 9.5,2.75 9,3.25 9,9.5
  pour Bottom (isolate 1.27): 1.25,99.25 178.25,99.25 178.25,2.75 0.75,2.75 0.75,99.25
I3  (via drill 0.8)
  Top 0.61: RV9.S 40.5,61.5 41.75,62.75 46.75,62.75 50,59.5 50,58.21 U6.2 | v65.75,73.5 73.5,81.25 86,81.25 89.5,77.75 89.5,75 88.25,73.75
  Top 0.813: 88.25,73.75 85.19,73.75 S2.2
  Bottom 0.61: U6.2 49.98,62.73 51.25,64 51.25,69.75 54.75,73.25 60.5,73.25 60.75,73.5 v65.75,73.5
I5  (via drill 0.8)
  Top 0.813: v68,73.25 68.25,73.25 73.25,78.25 82.48,78.25 S2.3
  Bottom 0.813: RV1.S 58.96,65.29 | 58.96,65.29 56.75,67.5 53.25,67.5 52.5,66.75 52.5,65.83 U6.6 | 58.96,65.29 60.04,65.29 v68,73.25
I12  (via drill 0.8)
  Top 0.61: RV8.S 120.25,60.75 121,60 144.42,60 U7.2 | v114.25,80 114,80 113.75,80.25 89.5,80.25 86.75,83 82.65,83 S2.4
  Bottom 0.61: RV8.S 119.71,74.54 v114.25,80
I-12
  Top 0.61: 115.25,81.5 117,79.75 117,72.5 120.75,68.75 145.83,68.75 U7.6 | 99.5,84.75 98,83.25 89.12,83.25 S2.5
  Top 0.813: 115.25,81.5 110.25,86.5 101.25,86.5 99.5,84.75
  Bottom 0.61: RV7.S 145.75,53.75 148,56 148,64.04 U7.6
IMAX
  Top 0.61: 55.06,65.44 U6.5 55.37,65.5 62.25,65.5 65.25,62.5 120.25,62.5 121.75,61 146.75,61 149.25,58.5 149.25,57.71 U7.3
  Bottom 0.61: 55.06,63.56 U6.5
  Bottom 0.813: 55.06,63.56 52.75,61.25 52.75,58.42 U6.3 52.5,58.17 52.5,57.5 49.72,54.72 X1.MP 47.5,52.03 RV2.2
N$1
  Bottom 0.813: U2.3 24.4,55.91 R1.2 24.56,52.52 R2.1
N$2
  Top 0.61: U2.2 21.86,58.86 23.25,60.25 30.31,60.25 R7.2
  Bottom 0.61: R8.1 R7.2
N$3
  Bottom 0.813: U2.6 24.75,66.41 24.75,67.25 28.81,71.31 R8.2 37.8,64.02 RV9.E
N$4
  Bottom 1.27: R27.2 101.75,55 99.5,52.75 99.5,47.53 R24.1
  Bottom 4: X7.2.MP X7.1.MP 99.17,6.08 R38.1 R37.1 R23.1 R24.1
N$5
  Bottom 0.813: U6.1 47.44,60.06 44.5,63 44.5,76.44 R9.1 46.08,79.52 U8.4
N$6
  Bottom 1.27: 56,47.25 56.58,47.25 R15.1 64.97,55.5 R16.2
  Bottom 4: X4.1.MP X4.2.MP 54.75,23.8 R12.1 R13.1 R14.1 56.65,40.94 R15.1
N$7
  Bottom 1.27: R18.2 83.89,51.69 R15.2
  Bottom 4: F2.2A 65,15.91 65,18 72.11,25.11 R12.2 R13.2 R14.2 87.81,46.59 R15.2
N$8
  Bottom 0.61: U3.3 74.27,57.54 R16.1
  Bottom 0.813: R16.1 R17.2
N$9
  Top 0.61: U3.2 71.73,58.48 73,59.75 80.06,59.75 R18.1
  Bottom 0.61: R19.2 80.5,60.19 80.06,59.75 R18.1
N$10
  Bottom 0.813: R19.1 78.56,71.31 74.5,67.25 74.5,66.04 U3.6 74.27,64.52 72.75,63 62.5,63 62,63.5 61.52,63.5 RV1.E
N$11
  Top 4: R38.2 111.59,25.34 108.25,22 108.25,21.5 108,21.25 108,16.91 F3.2A
  Bottom 1.27: R25.2 117.06,51.69 121.25,47.5 129.75,47.5 130,47.25 130.87,47.25 R24.2
  Bottom 4: R38.2 R37.2 R23.2 R24.2
N$12
  Bottom 0.813: U4.3 107.77,57.04 R27.1 R28.2
N$13
  Top 0.813: U4.2 105.23,58.48 106.5,59.75 113.56,59.75 R25.1
  Bottom 0.813: R26.2 R25.1
N$14
  Top 0.61: U4.6 107.81,65.56 108.5,66.25 109.25,67 112,67 112.5,66.5 119.5,66.5 122.25,63.75 RV8.E
  Bottom 0.61: R26.1 114,71.54 U4.6
N$15
  Bottom 0.61: U6.7 49.98,70.23 52.25,72.5 52.25,74.75 54.75,77.25 55.81,77.25 U8.10
  Bottom 0.813: 56.11,77.01 56.89,77.01 R20.1
  Bottom 1.27: 56.11,77.01 U8.10
N$16
  Bottom 0.61: U7.1 144.38,57.5 144.75,57.5 144.5,57.75 144.5,61.25 136.25,69.5 136.25,74.25 134.9,75.6 134.75,75.6 U9.4 130.61,79.12 R29.1
N$17
  Top 1.27: R34.2 140.61,29 R32.1
  Bottom 2.54: X10.1.MP 136.75,7.25 133.25,10.75 133.25,18.25 136.5,21.5 136.5,25.25 R32.1
N$18
  Bottom 0.813: U5.2 144.98,33.52 146.5,32 R33.2 148.81,31.75 R34.1
N$19
  Bottom 0.813: RV7.E 148.26,44.05 U5.6 147.75,43.08 147.75,42.5 146,40.75 143.25,40.75 140.5,38 140.5,33 141.44,32.06 R33.1
N$20
  Top 1.27: R35.2 154.42,29.69 R32.2
  Bottom 2.54: R32.2 159.29,24.04 158.5,23.25 158.5,15.59 F4.2A
N$21
  Bottom 0.813: U5.3 149.14,37.31 R35.1 R36.1
N$22
  Top 0.813: R39.2 160.5,51 165.01,51 RV5.3
N$23
  Bottom 0.813: R11.1 138.56,26.94 140.25,25.25 140.25,18.16 F4.1A
  Bottom 2.54: F4.1A 137.34,12.66 X10.2.MP
N$24
  Bottom 0.61: U7.7 146.73,65.52 145,67.25 145,73.25 141.38,76.88 | 141.38,76.88 141.25,77 138.65,77 U9.10 | R10.1 141.94,77.44 141.38,76.88
N$25
  Top 0.813: S2.13 79.79,76.05 X14.MP
N$26
  Bottom 0.61: S2.14 96.32,95.59 X17.MP
N$27
  Bottom 0.813: U11.2 132.23,55.54 R11.2 R40.1
N$29
  Top 0.813: LED1.A 43.41,72.16 45.75,74.5 48.4,74.5 U8.6
N$30
  Bottom 0.813: R21.1 40.49,75.1 LED1.K
N$31
  Top 0.61: U8.8 62.74,71.9 LED2.A
N$32
  Bottom 0.813: R22.1 63.1,74.8 LED2.K
N$33
  Bottom 1.27: X12.MP 168.75,8.75 178.75,18.75 178.75,30 177.25,31.5 Q1.2
N$35
  Bottom 0.61: U9.6 125.37,74.35 LED3.A
N$37
  Bottom 0.61: R30.1 121.78,76.6 LED3.K
N$38
  Top 0.61: LED4.A 139.14,72.41 U9.8
N$39
  Bottom 0.61: 146.29,75.02 LED4.K 144.96,76.35 R31.1
N$40
  Top 0.61: U9.5 131.14,76.89 135,80.75 156,80.75 156.75,80 158.78,80 U10.4
N$42
  Bottom 0.813: U10.6 U10.9 U10.10 166.54,77.5 167.25,77.5 168.5,78.75 168.5,81.25 167.26,82.49 U10.12 U10.13
N$44
  Bottom 1.27: R7.1 30.5,52.25 34.75,48 37.81,48 R6.2
  Bottom 4: F1.2A 20.09,19.59 25.25,24.75 38.09,24.75 R3.2 R4.2 R5.2 R6.2
N$45
  Bottom 1.27: R6.1 6.47,47.75 12.5,47.75 16.89,52.14 R2.2
  Bottom 2.54: 12.84,6.05 X1.1.MP
  Bottom 4: X1.2.MP 12.84,6.05 | X1.1.MP 12.84,18.36 R3.1 R4.1 R5.1 R6.1
Q1
  Bottom 1.27: Q1.1 176,62.78 U10.8
RESET
  Top 0.61: 56.9,84.6 U8.13 52.65,84.6 50.25,87 48.6,87 U8.1 | 131.5,87 130.97,87 U9.1 130.92,87.33 125,93.25 77,93.25 75.75,92
  Top 0.813: 56.9,84.6 68.35,84.6 75.75,92 | 131.5,87 134.75,87 137.25,84.5 U9.13 | U8.1 32.39,87.14 28.25,83 28.25,81.83 S1.1 S1.2
U8A
  Top 0.61: U8.5 52.23,76.98 53.5,78.25 64,78.25 70.25,84.5 | 129.25,85.75 133.5,85.75 136,83.25 152,83.25 156.32,87.57 U10.1 | 76,90 78,92 123,92 124.5,90.5
  Top 0.813: 70.25,84.5 70.5,84.5 76,90 | 124.5,90.5 129.25,85.75
U8B
  Top 0.61: U8.9 57.44,74.44 60,77 65.75,77 78.75,90 90.25,90 92.25,88 95.5,88 98,90.5 108.5,90.5 118.25,80.75 118.25,73 121.5,69.75 160,69.75 161.75,71.5 161.75,83.5 160.75,84.5
  Top 0.813: U10.2 160.22,85.03 160.75,84.5
U9B
  Top 0.61: U9.9 140.15,74.35 140.75,73.75 153,73.75 156.75,77.5 158.74,77.5 U10.5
